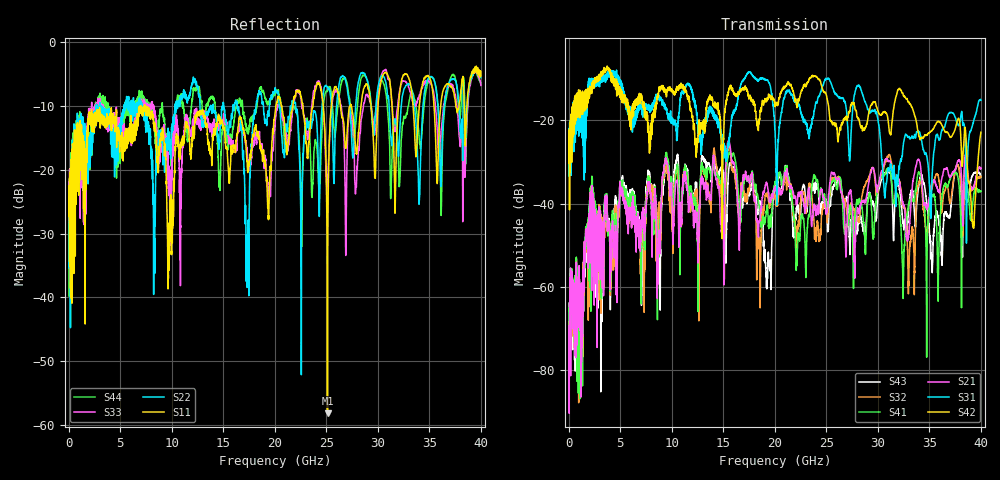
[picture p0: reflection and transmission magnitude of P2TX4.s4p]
!Agilent Technologies,N5245A,MY49151084,A.09.20.08
!Agilent N5245A: A.09.20.08
!Date: Thursday, March 01, 2012 14:07:50
!Correction: S11(Full 4 Port(1,2,3,4))
!S12(Full 4 Port(1,2,3,4))
!S13(Full 4 Port(1,2,3,4))
!S14(Full 4 Port(1,2,3,4))
!S21(Full 4 Port(1,2,3,4))
!S22(Full 4 Port(1,2,3,4))
!S23(Full 4 Port(1,2,3,4))
!S24(Full 4 Port(1,2,3,4))
!S31(Full 4 Port(1,2,3,4))
!S32(Full 4 Port(1,2,3,4))
!S33(Full 4 Port(1,2,3,4))
!S34(Full 4 Port(1,2,3,4))
!S41(Full 4 Port(1,2,3,4))
!S42(Full 4 Port(1,2,3,4))
!S43(Full 4 Port(1,2,3,4))
!S44(Full 4 Port(1,2,3,4))
!S4P File: Measurements: <S11,S12,S13,S14>,
!<S21,S22,S23,S24>,
!<S31,S32,S33,S34>,
!<S41,S42,S43,S44>:
# Hz S  dB  R 50
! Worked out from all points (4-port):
!   3996 points, 50 MHz to 40 GHz, reference 50 ohm
!   strongest paths, dB at 50 MHz, 10.04 GHz, 20.03 GHz, 30.02 GHz, 40 GHz:
!     S42: -26.5, -12.9, -16.6, -17.8, -22.9
!     S31: -25.0, -20.8, -22.5, -19.9, -15.2
!     S21: -69.4, -40.4, -36.0, -35.6, -31.6
!     S41: -68.0, -37.5, -34.7, -36.1, -37.1
!     S32: -66.8, -45.9, -38.5, -37.1, -33.5
!     S43: -63.9, -42.5, -35.0, -37.6, -33.6
!   lowest |S11| = -58.2 dB at 25.12 GHz (marker M1), VSWR 1.00, Z = 49.9 - j0.0331 ohm
!   |S11| at or under -10 dB: start of sweep to 7.01 GHz; 7.46 GHz to 20.11 GHz (12.65 GHz wide, 91.8 % of centre); 20.68 GHz to 21.76 GHz (1.072 GHz wide, 5.05 % of centre)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
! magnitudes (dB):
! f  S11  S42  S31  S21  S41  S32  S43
! 50 MHz  -24.3  -26.5  -25.0  -69.4  -68.0  -66.8  -63.9
! 9.44 GHz  -18.3  -13.7  -17.4  -29.2  -28.1  -30.6  -30.0
! 25.12 GHz  -58.2  -15.3  -10.0  -41.2  -40.5  -44.1  -45.9
! 30.71 GHz  -4.8  -18.0  -37.7  -29.5  -32.9  -30.1  -32.6
! 33.03 GHz  -5.8  -15.8  -23.9  -46.9  -40.0  -56.0  -40.2
! 39.24 GHz  -4.6  -44.9  -20.7  -36.1  -39.2  -36.4  -33.1
! 40 GHz  -5.3  -22.9  -15.2  -31.6  -37.1  -33.5  -33.6
